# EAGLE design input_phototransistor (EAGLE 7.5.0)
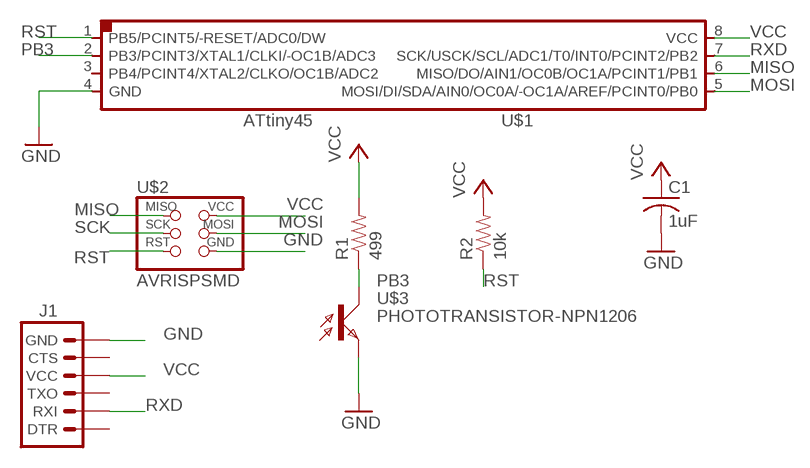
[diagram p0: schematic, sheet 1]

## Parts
C1  1uF  C-USC0805  [C0805]
J1  ARDUINO_SERIAL_PROGRAMSMD  [1X06-SMD]
R1  499  RESISTOR1206  [1206]
R2  10k  RESISTOR1206  [1206]
U$1  ATTINY45SI  [SOIC8]
U$2  AVRISPSMD  [2X03SMD]
U$3  PHOTOTRANSISTOR-NPN1206  [OP1206]

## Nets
GND: C1.2 J1.6(GND) U$1.4(GND) U$2.6(GND) U$3.EMITTER(E)
MISO: U$1.6(MISO/DO/AIN1/OC0B/OC1A/PCINT1/PB1) U$2.1(MISO)
MOSI: U$1.5(MOSI/DI/SDA/AIN0/OC0A/-OC1A/AREF/PCINT0/PB0) U$2.4(MOSI)
PB3: R1.1 U$1.2(PB3/PCINT3/XTAL1/CLKI/-OC1B/ADC3) U$3.COLLECTOR(C)
RST: R2.1 U$1.1(PB5/PCINT5/-RESET/ADC0/DW) U$2.5(RST)
RXD: J1.2(RXI) U$1.7(SCK/USCK/SCL/ADC1/T0/INT0/PCINT2/PB2)
SCK: U$2.3(SCK)
VCC: C1.1 J1.4(VCC) R1.2 R2.2 U$1.8(VCC) U$2.2(VCC)
Unconnected: J1.1(DTR) J1.3(TXO) J1.5(CTS) U$1.3(PB4/PCINT4/XTAL2/CLKO/OC1B/ADC2)

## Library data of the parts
C1 = rcl:C-US: CAPACITOR, American symbol
J1 = SparkFun-Connectors:ARDUINO_SERIAL_PROGRAM: FTDI connector footprints; PROD_ID: CONN-08971
R1 R2 = SparkFun-Passives:RESISTOR: Resistor
U$1 = fab:ATTINY45
U$2 = fab:AVRISP
U$3 = fab:PHOTOTRANSISTOR-NPN

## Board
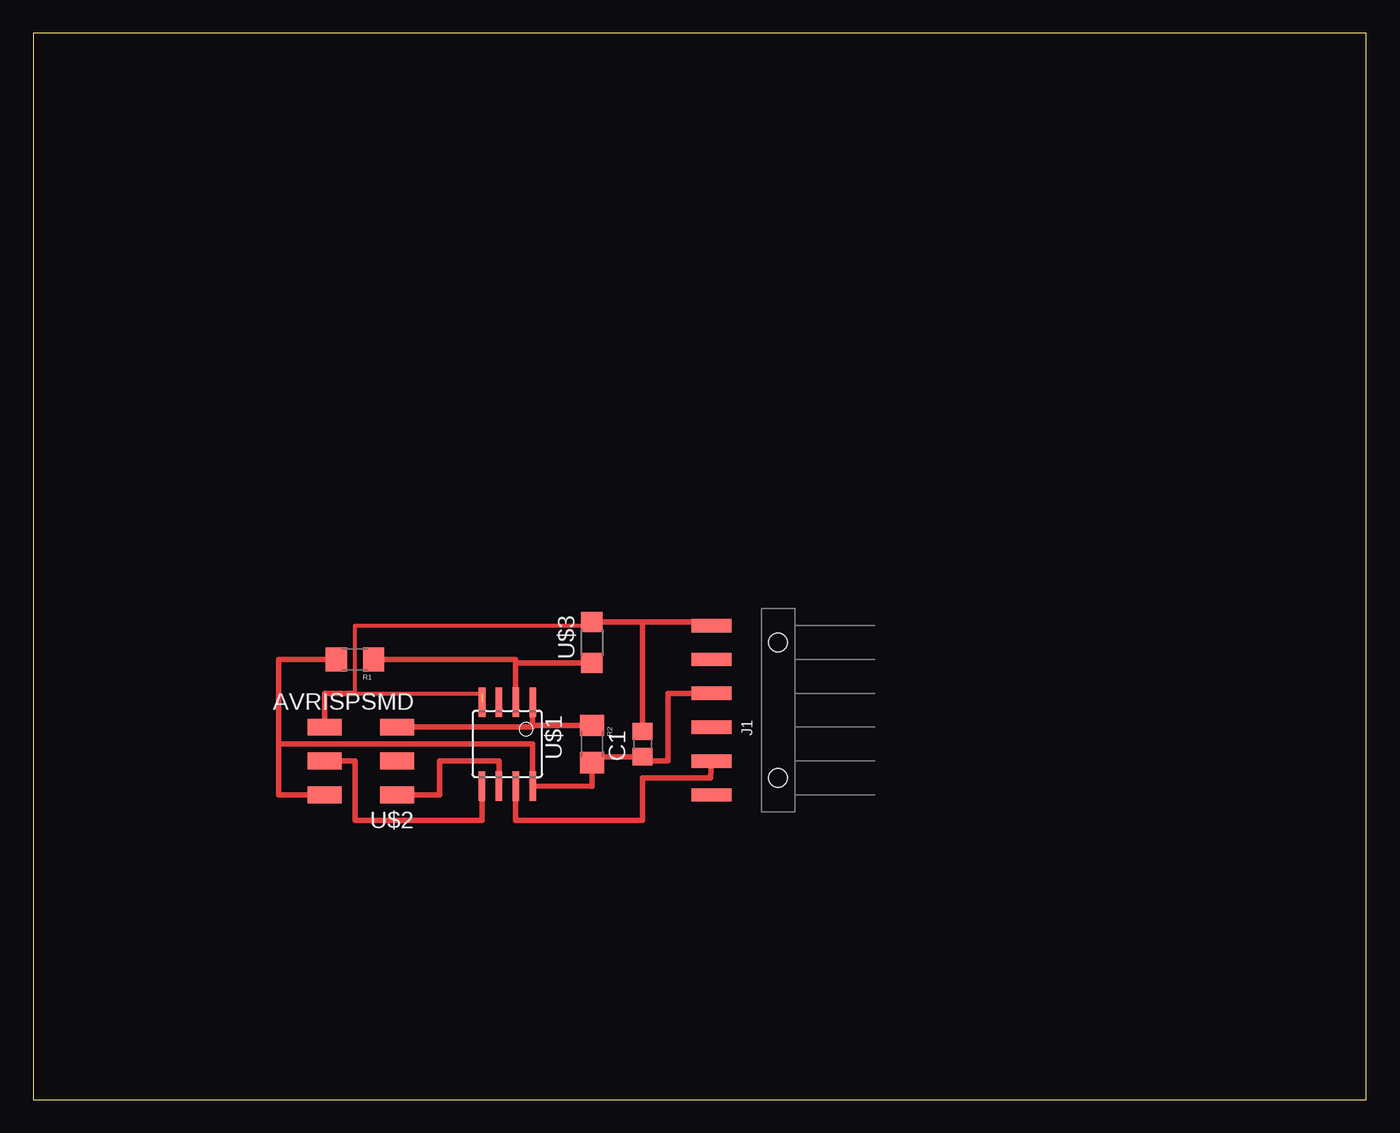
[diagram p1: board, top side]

Size 100 x 80 mm. Coordinates in mm from the lower left corner, seen from the top.
Outline: 0,0 100,0 100,80 0,80 0,0
Copper layers (1*16): Top 0.035mm / dielectric 1.5mm / Bottom 0.035mm
Design rules "default *": minimum track width 10mil, minimum drill 24mil, track to track 16mil, track to pad 16mil, pad to pad 16mil, via to via 16mil, smd to smd 16mil, copper to edge 40mil, drill to drill 8mil, minimum pad ring 10mil, minimum via ring 8mil, stop-mask expansion 4mil, vias tented up to drill 0mil, thermal gap 10mil

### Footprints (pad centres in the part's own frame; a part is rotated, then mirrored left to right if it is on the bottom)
C0805 = smd 1.3 x 1.5: 1 -0.95,0; 2 0.95,0
1X06-SMD = smd 1 x 3: 1 -6.35,5; 2 -3.81,5; 3 -1.27,5; 4 1.27,5; 5 3.81,5; 6 6.35,5 | hole 1.4: -5.08,0; 5.08,0
1206 = smd 1.6 x 1.8: 1 -1.4,0; 2 1.4,0
SOIC8 = smd 0.5 x 2.2: 1 -1.905,-3.154; 2 -0.645,-3.154; 3 0.625,-3.154; 4 1.895,-3.154; 5 1.905,3.154; 6 0.635,3.154; 7 -0.635,3.154; 8 -1.905,3.154
2X03SMD = smd 2.54 x 1.27: 1 -2.54,2.54; 2 2.92,2.54; 3 -2.54,0; 4 2.92,0; 5 -2.54,-2.54; 6 2.92,-2.54
OP1206 = smd 1.5 x 1.6: COLLECTOR -1.55,0; EMITTER 1.55,0

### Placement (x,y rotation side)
C1  45.72,26.67 90 top
J1  55.88,29.21 90 top
R1  24.13,33.02 180 top
R2  41.91,26.67 270 top
U$1  35.56,26.67 180 top
U$2  24.77,25.4 180 top
U$3  41.91,34.29 90 top

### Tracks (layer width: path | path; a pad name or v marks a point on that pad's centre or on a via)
GND  (2 unrouted)
  Top 0.305: U$3.EMITTER 41.91,35.56 24.13,35.56 24.13,30.48 33.66,30.48
  Top 0.406: U$1.4 | U$3.EMITTER 45.72,35.84 | 45.72,35.84 50.88,35.84 J1.6 | C1.2 45.72,35.84 | 24.13,30.48 21.84,30.48 U$2.6
MISO
  Top 0.406: U$1.6 34.92,25.4 30.48,25.4 30.48,22.86 U$2.1
MOSI
  Top 0.406: U$2.4 24.13,25.4 24.13,20.95 33.66,20.95 U$1.5
PB3
  Top 0.406: R1.1 36.2,33.02 36.2,32.74 | 36.2,32.74 36.2,30.48 U$1.2 | U$3.COLLECTOR 36.2,32.74
RST
  Top 0.406: R2.1 37.47,28.07 | 37.47,28.07 37.47,27.94 U$2.5 | U$1.1 37.47,28.07
RXD
  Top 0.406: J1.2 50.8,24.13 45.72,24.13 45.72,20.95 36.2,20.95 U$1.7
VCC
  Top 0.406: R1.2 18.41,33.02 18.41,26.67 | 18.41,26.67 18.41,22.86 U$2.2 | J1.4 47.62,30.48 47.62,25.4 45.72,25.4 C1.1 41.91,25.72 R2.2 41.91,23.5 U$1.8 37.47,26.67 18.41,26.67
